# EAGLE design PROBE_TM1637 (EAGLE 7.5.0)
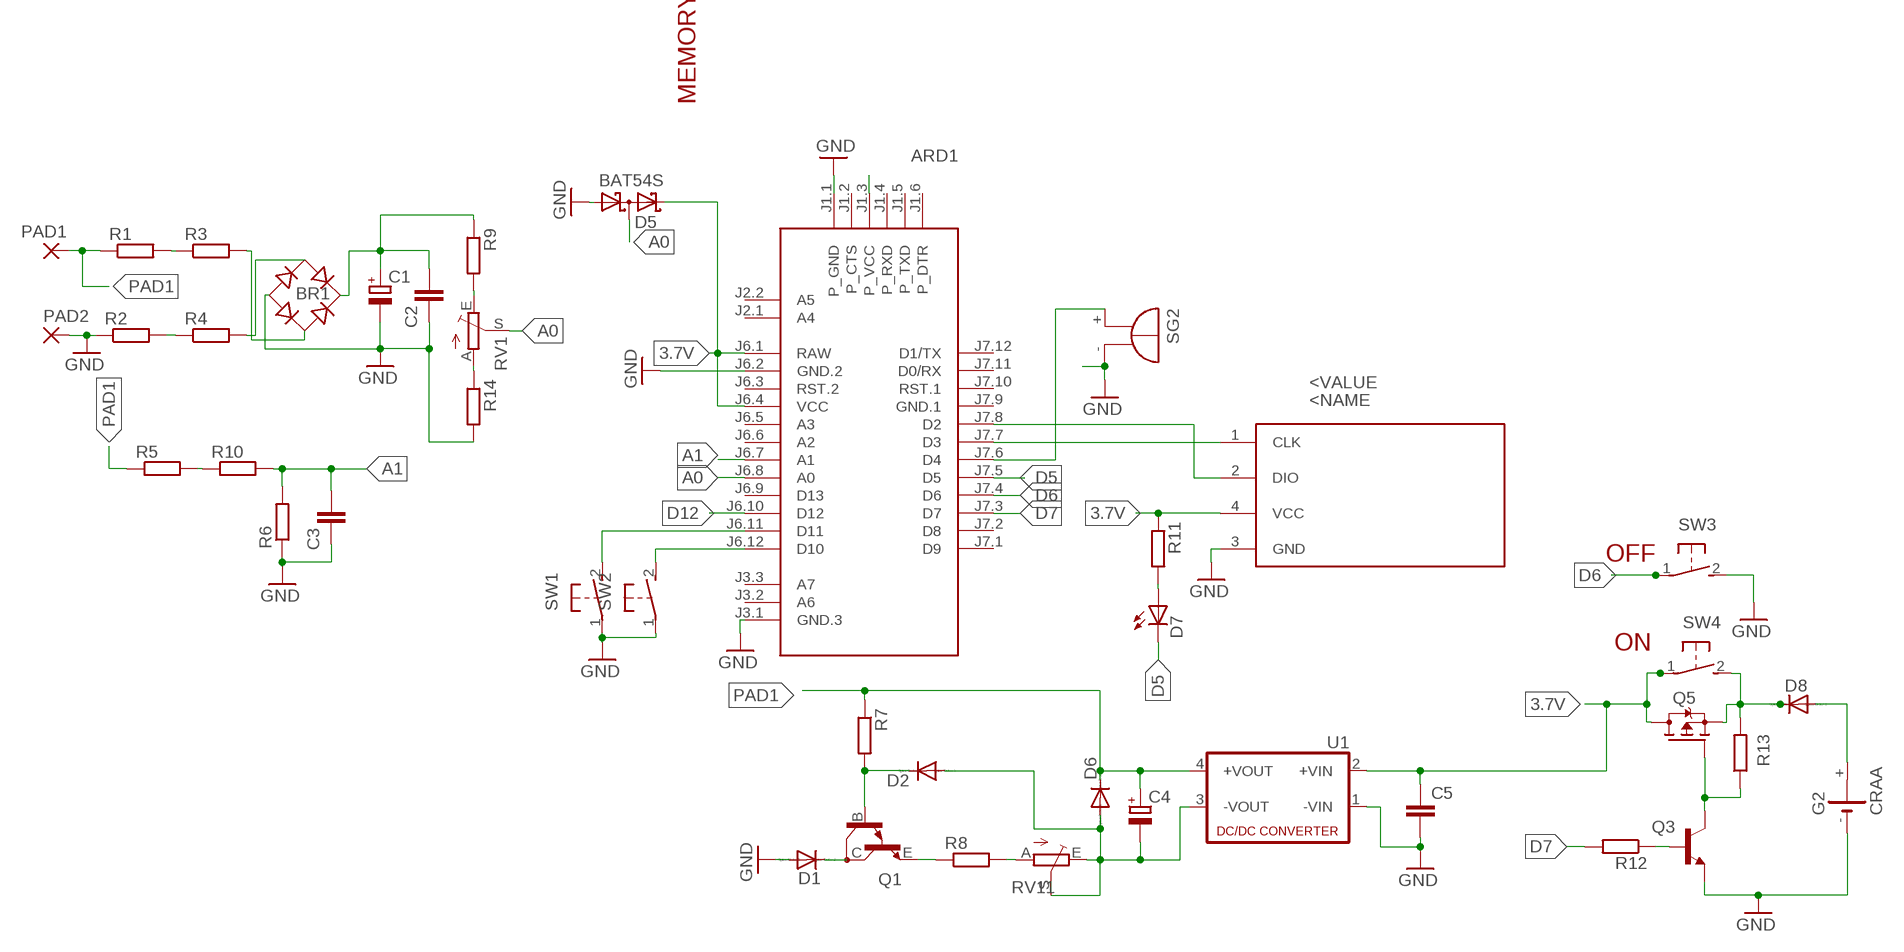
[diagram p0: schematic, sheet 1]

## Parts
ARD1  ARDUINO-PRO-MINI-3.3V  [ARDUINO-PRO-MINI]
BR1  DBL208G  [DB]
C1  CPOL-EUD/7343-31W  [D/7343-31W]
C2  C-EUC1206  [C1206]
C3  C-EUC1206  [C1206]
C4  CPOL-EUC/6032-28R  [C/6032-28R]
C5  C-EUC1206  [C1206]
D1  CGRM4007-G  [SOD-123_MINI-SMA]
D2  CGRM4001-G  [SOD-123_MINI-SMA]
D5  BAT54S  [SOT23]
D6  CGRM4001-G  [SOD-123_MINI-SMA]
D7  LED3MM  [LED3MM]
D8  CGRM4007-G  [SOD-123_MINI-SMA]
DIS1  TM1637  [TM1637]
G2  CRAA  [CRAA]
PAD1  3,81/1,1  [3,81/1,1]
PAD2  3,81/1,1  [3,81/1,1]
Q1  BDV65  [SOT93]
Q3  BC818-16SMD  [SOT23-BEC]
Q5  BSP170P  [SOT223]
R1  R-EU_R2512  [R2512]
R2  R-EU_R2512  [R2512]
R3  R-EU_R2512  [R2512]
R4  R-EU_R2512  [R2512]
R5  R-EU_R2512  [R2512]
R6  R-EU_R2512  [R2512]
R7  R-EU_R2512  [R2512]
R8  R-EU_R2010  [R2010]
R9  R-EU_R0805  [R0805]
R10  R-EU_R2512  [R2512]
R11  R-EU_R0805  [R0805]
R12  R-EU_R0805  [R0805]
R13  R-EU_R0805  [R0805]
R14  R-EU_R0805  [R0805]
RV1  TRIM_EU-CT6  [CT6]
RV11  TRIM_EU-CT6  [CT6]
SG2  BMT1205XH7.5  [BMT1205XH7.5]
SW1  31-XX  [B3F-31XX]
SW2  31-XX  [B3F-31XX]
SW3  31-XX  [B3F-31XX]
SW4  31-XX  [B3F-31XX]
U1  NME  [NME]

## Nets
3.7V: ARD1.J6.1(RAW) ARD1.J6.4(VCC) C5.1 D5.2(C2) DIS1.4(VCC) Q5.2(D) Q5.4(D) R11.1 SW4.1(P) U1.2(+VIN)
A0: ARD1.J6.8(A0) D5.3(C1A2) RV1.S
A1: ARD1.J6.7(A1) C3.2 R6.2 R10.2
D5: ARD1.J7.5(D5) D7.K(C)
D6: ARD1.J7.4(D6) SW3.1(P)
D7: ARD1.J7.3(D7) R12.2
D12: ARD1.J6.10(D12)
GND: ARD1.J1.1(P_GND) ARD1.J3.1(GND.3) ARD1.J6.2(GND.2) BR1.- C1.- C2.1 C3.1 C5.2 D1.A D5.1(A1) DIS1.3(GND) G2.- PAD2.1(P) Q3.E R2.1 R6.1 R14.2 SG2.- SW1.1(P) SW2.1(P) SW3.2(S) U1.1(-VIN)
N$1: BR1.AC1 R4.2
N$2: R1.2 R3.1
N$3: R2.2 R4.1
N$4: BR1.AC2 R3.2
N$5: BR1.+ C1.+ C2.2 R9.1
N$6: R9.2 RV1.E
N$7: R14.1 RV1.A
N$8: Q1.E R8.1
N$9: R8.2 RV11.A
N$10: C4.- D2.A D6.A RV11.E RV11.S U1.3(-VOUT)
N$11: D8.A G2.+
N$12: D1.C Q1.C
N$13: R5.2 R10.1
N$14: ARD1.J7.7(D3) DIS1.1(CLK)
N$15: D8.C Q5.3(S) R13.2 SW4.2(S)
N$16: Q3.C Q5.1(G) R13.1
N$17: ARD1.J7.8(D2) DIS1.2(DIO)
N$18: Q3.B R12.1
N$19: ARD1.J1.3(P_VCC)
N$20: D2.C Q1.B R7.2
N$21: D7.A R11.2
N$22: ARD1.J6.11(D11) SW1.2(S)
N$23: ARD1.J6.12(D10) SW2.2(S)
N$24: ARD1.J7.6(D4) SG2.+
PAD1: C4.+ D6.C PAD1.1(P) R1.1 R5.1 R7.1 U1.4(+VOUT)
Unconnected: ARD1.J1.2(P_CTS) ARD1.J1.4(P_RXD) ARD1.J1.5(P_TXD) ARD1.J1.6(P_DTR) ARD1.J2.1(A4) ARD1.J2.2(A5) ARD1.J3.2(A6) ARD1.J3.3(A7) ARD1.J6.3(RST.2) ARD1.J6.5(A3) ARD1.J6.6(A2) ARD1.J6.9(D13) ARD1.J7.1(D9) ARD1.J7.2(D8) ARD1.J7.10(RST.1) ARD1.J7.11(D0/RX) ARD1.J7.12(D1/TX) G2.+@1(+)

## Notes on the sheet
- MEMORY
- OFF
- ON

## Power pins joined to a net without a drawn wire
GND.1: ARD1.J7.9(GND.1)

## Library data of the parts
ARD1 = diy-modules:ARDUINO-PRO-MINI-*: Arduino Pro Mini and compatible devices More details available here: https://www.arduino.cc/en/Main/ArduinoBoardProMini Click here to find device on ebay.com
BR1 = rectifier:DB?*G: Single Phase 1.0 AMP Glass Passivated Bridge Rectifier Taiwan Semiconductor Co.,Ltd. - TSC Source: http://www.taiwansemi.com/TSCbig5/ezcatfiles/cust/img/img/db101g.pdf http://www.ts.com.tw/db/pictures/modules/PDT/PDT060207001/DBLS201G.pdf
C1 C4 = rcl:CPOL-EU: POLARIZED CAPACITOR, European symbol
C2 C3 C5 = rcl:C-EU: CAPACITOR, European symbol
D1 D2 D6 D8 = diode:CGRM400*-G: Molded plasitc,JEDEC SOD-123/Mini SMA
D5 = diode:BAT54S: Schottky Diodes Pin connection corrected 2011-05-04 Source: Fairchild .. BAT54.pdf
D7 = led:LED: LED
DIS1 = diy-modules:TM1637
G2 = battery:CRAA: LI BATTERY Varta
PAD1 PAD2 = wirepad:3,81/1,1: THROUGH-HOLE PAD
Q1 = transistor:BDV65: NPN BIPOLAR DARLINGTON TRANSISTOR
Q3 = transistor-npn:BC818*: NPN Transistor
Q5 = transistor-fet:BSP170P: SIPMOS(R) Small-Signal-Transistor P-Channel, Enhancement mode Source: http://www.infineon.com/upload/Document/BSP170P_Rev2.4.pdf
R1-R14 = rcl:R-EU_: RESISTOR, European symbol
RV1 RV11 = pot:TRIM_EU-: POTENTIOMETER
SG2 = buzzer:BMT1205XH7.5: MAGNETIC TRANSDUCER; OC_FARNELL: unknown; OC_NEWARK: unknown
SW1-SW4 = switch-omron:31-XX: OMRON SWITCH; MPN: B3F-3100; OC_FARNELL: 959704; OC_NEWARK: 36M3582
U1 = dc-dc-converter:NME: DC-DC CONVERTER; MF: C & D TECHNOLOGIES, INC; MPN: NME1205D; OC_FARNELL: 1021466; OC_NEWARK: 98B8198

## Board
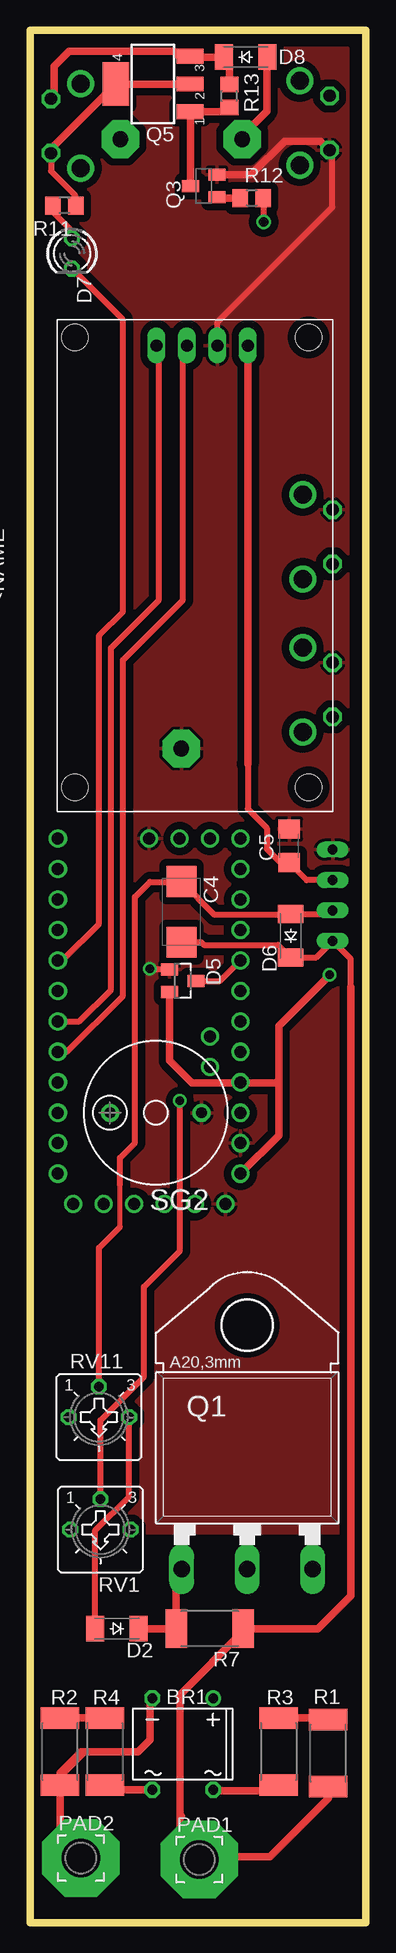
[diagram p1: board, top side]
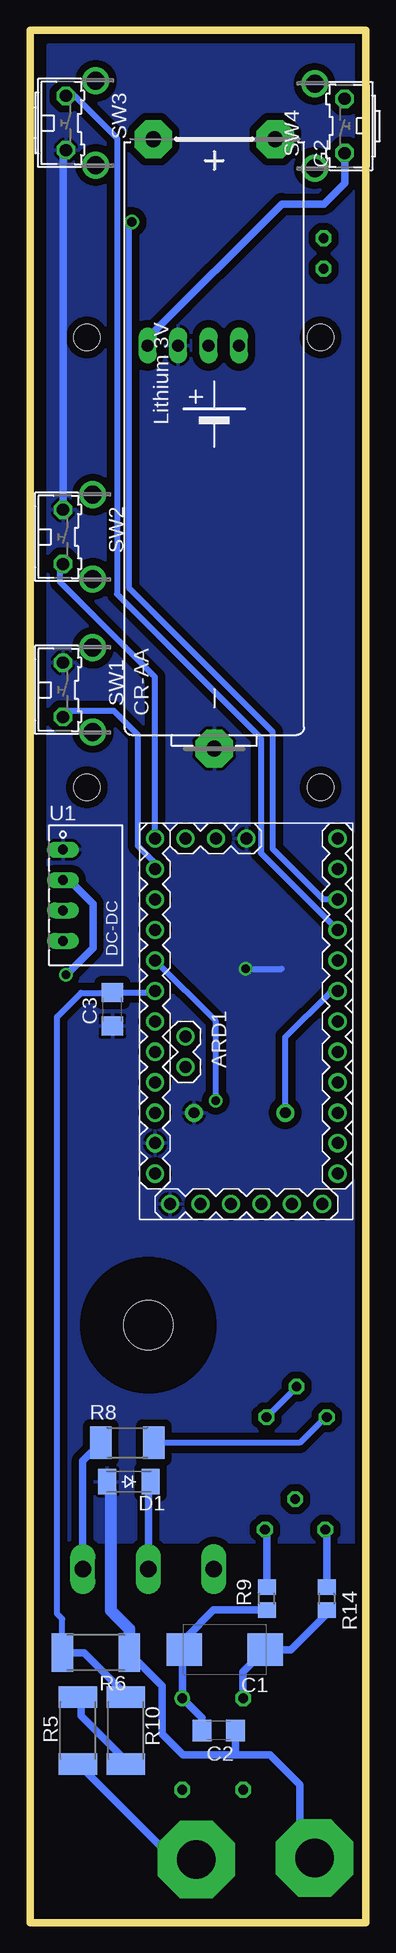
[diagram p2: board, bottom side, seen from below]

Size 28 x 157.75 mm. Coordinates in mm from the lower left corner, seen from the top.
Outline: 0,0 28,0 28,157.75 0,157.75 0,0
Copper layers (1*16): Top 0.035mm / dielectric 1.5mm / Bottom 0.035mm
Design rules "default *": minimum track width 10mil, minimum drill 24mil, track to track 8mil, track to pad 8mil, pad to pad 8mil, via to via 8mil, smd to smd 8mil, copper to edge 20mil, drill to drill 8mil, minimum pad ring 10mil, minimum via ring 8mil, stop-mask expansion 4mil, vias tented up to drill 0mil, thermal gap 10mil

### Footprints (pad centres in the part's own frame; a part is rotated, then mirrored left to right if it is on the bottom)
ARDUINO-PRO-MINI = drill 1: J1.1 -15.24,6.35; J1.2 -15.24,3.81; J1.3 -15.24,1.27; J1.4 -15.24,-1.27; J1.5 -15.24,-3.81; J1.6 -15.24,-6.35; J2.1 -1.27,5.08; J2.2 -3.81,5.08; J3.1 15.24,0; J3.2 15.24,2.54; J3.3 15.24,5.08; J6.1 -12.7,7.62; J6.2 -10.16,7.62; J6.3 -7.62,7.62; J6.4 -5.08,7.62; J6.5 -2.54,7.62; J6.6 0,7.62; J6.7 2.54,7.62; J6.8 5.08,7.62; J6.9 7.62,7.62; J6.10 10.16,7.62; J6.11 12.7,7.62; J6.12 15.24,7.62; J7.1 15.24,-7.62; J7.2 12.7,-7.62; J7.3 10.16,-7.62; J7.4 7.62,-7.62; J7.5 5.08,-7.62; J7.6 2.54,-7.62; J7.7 0,-7.62; J7.8 -2.54,-7.62; J7.9 -5.08,-7.62; J7.10 -7.62,-7.62; J7.11 -10.16,-7.62; J7.12 -12.7,-7.62
DB = drill 0.813: + -2.54,-3.81 | drill 0.813 octagon: - 2.54,-3.81; AC1 2.54,3.81; AC2 -2.54,3.81
D/7343-31W = smd 2.95 x 2.7: + 3.375,0; - -3.375,0
C1206 = smd 1.6 x 1.8: 1 -1.4,0; 2 1.4,0
C/6032-28R = smd 2.55 x 2.5: + 2.525,0; - -2.525,0
SOD-123_MINI-SMA = smd 1.5 x 2.1: A 1.8,0; C -1.8,0
SOT23 = smd 1 x 1.4: 1 -0.95,-1.1; 2 0.95,-1.1; 3 0,1.1
LED3MM = drill 0.813 octagon: A -1.27,0; K 1.27,0
TM1637 = drill 1 long: 1 36.83,12.7; 2 36.83,10.16; 3 36.83,7.62; 4 36.83,5.08 | hole 2.2: 0,0; 37.5,0; 0,19.5; 37.5,19.5
CRAA = drill 1.321 pad 3.15 octagon: + -25.4,-5.08; +@1 -25.4,5.08; - 25.4,0
3,81/1,1 = drill 3.2 pad 6.452 octagon: 1 0,0
SOT93 = drill 1.397 long: B -5.461,-10.16; C 0,-10.16; E 5.461,-10.16 | hole 4.115: 0,10.16
SOT23-BEC = smd 1 x 1.4: B -0.95,-1.1; C 0,1.1; E 0.95,-1.1
SOT223 = smd 1.219 x 2.235: 1 -2.311,-3.099; 2 0,-3.099; 3 2.311,-3.099 | smd 3.6 x 2.2: 4 0,3.099
R2512 = smd 1.8 x 3.2: 1 -2.8,0; 2 2.8,0
R2010 = smd 1.8 x 2.7: 1 -2.2,0; 2 2.2,0
R0805 = smd 1.3 x 1.5: 1 -0.95,0; 2 0.95,0
CT6 = drill 0.813 octagon: A 2.515,0; E -2.515,0; S 0,-2.54
BMT1205XH7.5 = drill 0.9 pad 1.5: + 3.8,0; - -3.8,0
B3F-31XX = drill 1.016 octagon: 1 -2.261,-1.245; 2 2.261,-1.245 | drill 1.499 pad 2.159: 3 -3.505,1.245; 4 3.505,1.245
NME = drill 0.813 long: 1 0,3.81; 2 0,1.27; 3 0,-1.27; 4 0,-3.81

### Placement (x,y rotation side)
ARD1  9.95,75.12 90 bottom
BR1  12.75,14.88 180 top
C1  11.75,22.75 180 bottom
C2  12.25,16 180 bottom
C3  21.12,76.12 90 bottom
C4  12.62,84.25 270 top
C5  21.62,89.75 90 top
D1  19.75,36.75 180 bottom
D2  7.25,24.5 180 top
D5  12.75,78.5 270 top
D6  21.75,82.25 90 top
D7  3.5,139.12 270 top
D8  18,155.5 0 top
DIS1  23.25,94.62 90 top
G2  12.62,123.25 270 bottom
PAD1  14.12,5.25 0 top
PAD2  4.25,5.38 0 top
Q1  18.12,39.62 0 top
Q3  14.5,144.75 90 top
Q5  10.25,153.25 90 top
R1  24.88,14.12 90 top
R2  2.5,14.25 90 top
R3  20.75,14.25 270 top
R4  6.25,14.25 270 top
R5  24,16 90 bottom
R6  22.5,22.5 180 bottom
R7  15,24.5 180 top
R8  19.88,40 0 bottom
R9  8.25,27 90 bottom
R10  20,16 90 bottom
R11  2.88,143.12 180 top
R12  18.5,143.75 0 top
R13  16.62,152.25 90 top
R14  3.25,27 270 bottom
RV1  5.88,32.75 180 top
RV11  5.75,42.12 180 top
SG2  10.5,67.5 180 top
SW1  24,102.75 270 bottom
SW2  24,115.5 270 bottom
SW3  23.75,150 270 bottom
SW4  3,149.75 90 bottom
U1  25.25,85.62 0 bottom

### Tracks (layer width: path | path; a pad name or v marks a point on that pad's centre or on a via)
3.7V  (via drill 0.7)
  Top 0.5: SW4.1 1.75,146 3.75,144 3.75,143.2 R11.1 | 18.17,96.58 18.17,92.83 19.75,91.25 19.75,89.5 21,88.25 21.52,88.25 C5.1 23.08,86.89 U1.2
  Top 0.61: SW4.1 1.75,147.85 Q5.4 Q5.2 | DIS1.4 18.17,96.58 | D5.2 11.65,71.85 13.5,70 17.53,70 | 17.53,70 ARD1.J6.4 | ARD1.J6.1 20.75,65.6 20.75,70.25 | 20.75,70.25 20.75,74.75 v25,79 | 17.53,70 20.5,70 20.75,70.25
  Bottom 0.61: DIS1.4 18.17,132.08 7,143.25 3.5,143.25 1.75,145 SW4.1 | v25,79 22.75,81.25 22.75,84.89 24.75,86.89 U1.2
A0  (via drill 0.7 pad 0.61)
  Top 0.5: D5.3 15.87,78.5 ARD1.J6.8 | RV1.S 5.88,41.88 9.5,45.5 9.5,53 12.5,56 v12.5,68.5
  Bottom 0.5: v12.5,68.5 12.5,75.13 ARD1.J6.8
A1
  Bottom 0.5: R6.2 25.3,25.3 25.75,25.75 25.75,75.5 23.75,77.5 21.15,77.5 C3.2 17.7,77.53 ARD1.J6.7
  Bottom 0.61: R10.2 20,19 23.5,22.5 R6.2
D5
  Top 0.5: ARD1.J7.5 2.6,80.2 arc45 2.77,80.27 5.75,83.25 5.75,107.14 arc-45 5.82,107.32 7.75,109.25 7.75,133.5 arc45 7.68,133.68 D7.K
D6
  Bottom 0.5: SW3.1 24.26,152.26 20.75,148.75 20.75,110.75 8.75,98.75 8.75,89.16 ARD1.J7.4
D7  (via drill 0.8)
  Top 0.5: v19.5,141.75 19.5,143.7 R12.2
  Bottom 0.5: ARD1.J7.3 3.53,85.28 7.75,89.5 7.75,99.25 19.75,111.25 19.75,141.5 v19.5,141.75
GND  (via drill 0.7 pad 0.61)
  Top 0.5: DIS1.3 15.63,133.38 25.25,143 25.25,147.49 SW3.2 | D5.1 10.55,79.45 v10,79.5
  Top 0.61: Q3.E 18.45,145.7 21.25,148.5 24.23,148.5 SW3.2 | 2.5,12.25 R2.1 2.5,7.12 PAD2.1 | 2.5,12.25 2.5,12.5 4.25,14.25 4.5,14.25 | BR1.- 10,18.4 10,15.25 9,14.25 4.5,14.25 | 4.5,14.25 2.5,12.25
  Bottom 0.5: v10,79.5 7,79.5
  Bottom 0.61: SW2.1 25.25,147.49 SW3.2 | R6.1 19.7,22.45 17,19.75 17,15.75 15.25,14 10.75,14 | 10.75,14 8,14 5.5,11.5 5.5,6.62 PAD2.1 | C2.1 10.85,14.1 10.75,14 | BR1.- 10.21,20.91 C1.- 6.25,22.75 3.25,25.75 R14.2
  Bottom 1.016: R6.1 19.7,24.45 21.25,26 21.25,36 21.5,36.25
  pour Bottom (isolate 0.61): 0.5,156.5 26.5,156.5 26.5,31.75 0.5,31.75
  pour Top (isolate 0.61): 1,156.25 26.5,156.25 26.5,32.5 1,32.5
N$1
  Top 0.61: BR1.AC1 6.63,11.07 R4.2
N$2
  Top 0.61: R3.1 24.2,17.05 24.25,17 24.8,17 R1.2
N$3
  Top 0.61: R4.1 3.45,17.05 3.25,17.25 2.7,17.25 R2.2
N$4
  Top 0.61: R3.2 19.7,11.45 19.25,11 15.36,11 BR1.AC2
N$5
  Bottom 0.61: R9.1 12.7,26.05 15,23.75 15,22.88 C1.+ | 14.79,22.41 C1.+ | C2.2 13.65,17.05 BR1.+ 15.29,22.59 C1.+
N$6
  Bottom 0.61: R9.2 8.25,32.61 RV1.E
N$7
  Bottom 0.61: R14.1 3.25,32.64 RV1.A
N$8
  Bottom 0.61: Q1.E 23.59,38.49 R8.1
N$9
  Bottom 0.5: RV11.A 3.38,42.12 5.5,40 R8.2
N$10
  Top 0.406: 7.5,58 7.5,61.5
  Top 0.5: D2.A 5.45,32.7 8.25,35.5 RV11.E | RV11.S 5.75,56.25 7.5,58 | 8.75,76.75 8.75,85.5 10,86.75 12.6,86.75 C4.- 15.4,84 21.7,84 D6.A 24.95,84.05 U1.3
  Top 0.506: 7.5,61.5 7.5,63.75 8.75,65 8.75,76.75
  Bottom 0.5: RV11.S 5.75,44.64 RV11.E
N$11
  Top 0.61: G2.+ 17.7,148.96 19.75,151 19.75,155.45 D8.A
N$12
  Bottom 0.61: Q1.C 18.12,36.58 D1.C
N$13
  Bottom 0.61: R10.1 20,13.5 23.75,17.25 23.75,18.55 R5.2
N$14
  Top 0.5: ARD1.J7.7 4.12,75.12 6.75,77.75 6.75,106.25 10.75,110.25 10.75,131.25 DIS1.1
N$15
  Top 0.61: R13.2 16.62,155.07 D8.C 13.41,155.5 Q5.3 12.44,155.56 12,156 3.25,156 2,154.75 2,152.25 SW4.2
N$16
  Top 0.61: Q3.C 13.4,150.89 Q5.1 16.26,150.94 R13.1
N$17
  Top 0.5: ARD1.J7.8 3.08,72.58 7.75,77.25 7.75,105.25 12.75,110.25 12.75,131.12 DIS1.2
N$18
  Top 0.61: R12.1 15.65,143.75 Q3.B
N$20
  Top 0.61: Q1.B 12.2,29 R7.2 D2.C
N$21
  Top 0.5: D7.A 3.5,141 2,142.5 2,143.05 R11.2
N$22
  Bottom 0.5: ARD1.J6.11 17.57,88.22 arc-45 17.64,88.39 19,89.75 19,98.89 arc-45 19.07,99.07 20.75,100.75 | 24.88,100.75 arc-45 25.06,100.68 SW1.2
  Bottom 0.506: 20.75,100.75 21,101 24.73,101 SW1.2
N$23
  Bottom 0.5: ARD1.J6.12 17.57,103.82 25.5,111.75 25.5,112.98 SW2.2
N$24
  Bottom 0.506: SG2.+ 6.7,73.8 3,77.5 2.49,77.5 ARD1.J7.6
PAD1
  Top 0.5: C4.+ 14.28,81.72 14.5,81.5 20.7,81.5 D6.C 23.89,80.45 U1.4 26.75,80.31 26.75,78
  Top 0.61: 12.5,8.75 12.5,19 17.8,24.3 R7.1 24,24.5 26.75,27.25 26.75,78 | 12.5,8.75 12.5,7.5 14.25,5.75 14.25,5.38 PAD1.1 14.38,5.5 20,5.5 24.88,10.38 R1.1 | 12.62,8.88 12.5,8.75
  Bottom 0.61: R5.1 23.95,13.2 16.25,5.5 14.38,5.5 PAD1.1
